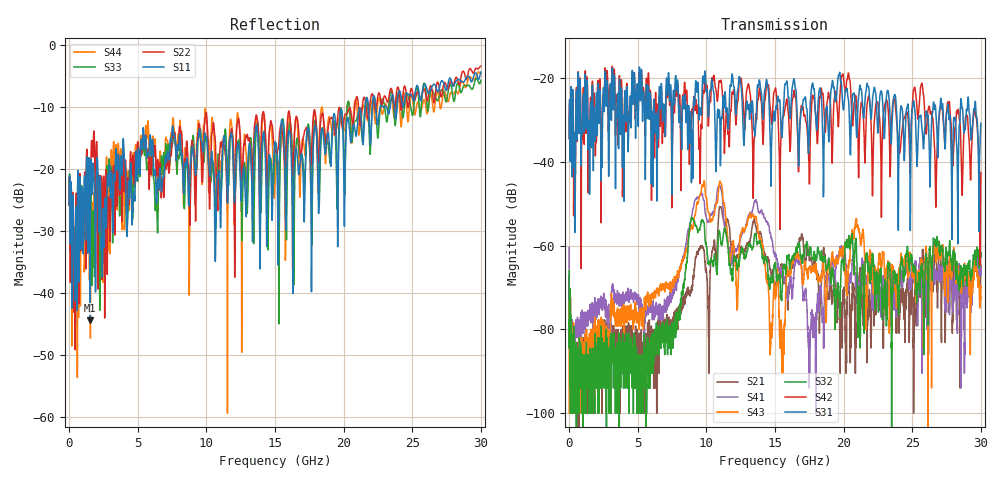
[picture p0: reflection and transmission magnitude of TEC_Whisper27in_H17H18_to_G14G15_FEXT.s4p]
! Tyco Electronics
! H17H18-G14G15_FEXT
!! PART DESCRIPTION: Whisper 27in Megtron 6 VLP-HVLP-VLP Channel Model, bulkhead 2.4mm test pts
!! MODEL DESCRIPTION: System 4-port S-parameter
!! MODEL STATUS: Measured
!! MODEL GEOMETRY: Channel Model
!! MODEL FREQUENCY RANGE: DC to 30.000 GHz in 10.000 MHz frequency steps
!! MODEL EDGE RATE LIMITATION: 12.500 ps (Using conservative 0.5/Fmax rule of thumb)
!! TIME-DOMAIN TRANSFORM CAUTIONS:
!! 1.) Do not simulate transient edge rates faster than the number listed above.  Edge rates faster than this number
!!  contain significant spectral content at frequencies above the model's highest frequency.
!! 2.) Even when simulating edge rates that are slower than the number listed above, be aware that the best time
!!  resolution possible with a direct iFFT is (1 / 2Fmax).  As a result, time resolution is typically not adequate
!!  for most time-domain simulations unless tricks such as windowing are used to minimize leakage and aliasing.
!! 3.) Because the model has a uniform frequency step, a direct iFFT will result in an impulse that that has a time
!!  length given by either (1 / Fstep) or (1 / 2Fstep), depending on the transform being used.  Care has been taken
!!  in selecting the frequency step to ensure a settled impulse response for the model.  Therefore, convolution with
!!  the model's impulse response should present no issues.  However, if directly concatenating s-parameter models
!!  in the frequency domain a user must either interpolate necessary interim frequencies or complete impulse response
!!  zero-padding.  Impulse response zero-padding is more difficult, but more accurate.
!! PORT DEFINITIONS:
!! Port  1  ----->  Side A  H17  G14  Side B  <-----  Port  2
!! Port  3  ----->  Side A  H18  G15  Side B  <-----  Port  4
! Point-to-Point link (differential)  !
! Connectors:  !
!  1: STRADA Whisper  !
! Materials:  !
!  Backplane: Megtron-6 HVLP  !
!  Daughtercard: Megtron-6 VLP  !
! Stack-up:  !
!  Backplane: 20 layers, 200mil thick  !
!  Daughtercard: 14 layers, 110mil thick  !
! Trace Length:  !
!  Backplane: 17in  !
!  Daightercards: 5in  !
! Trace Width:  !
!  Backplane: 8-13-8 mils  !
!  Daughtercards: 6-9-6 mils  !
! Geometry:  !
!  Backplane: Stripline  !
!  Daughtercards: Stripline  !
! Freq. Range: 0 GHz - 30 GHz  !
! Note1: non-mixed-mode s-parameters  !
! Note2: channel includes 2.4mm test points  !
! Touchstone data converted from IdEM dataset
# GHz S MA R 50
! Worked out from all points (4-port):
!   3000 points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, 10 MHz to 30 GHz, reference 50 ohm
!   strongest paths, dB at 10 MHz, 7.51 GHz, 15.01 GHz, 22.51 GHz, 30 GHz:
!     S31: -34.4, -43.9, -30.2, -32.7, -30.8
!     S42: -34.5, -40.8, -22.7, -26.3, -42.6
!     S32: -66.0, -80.0, -64.9, -71.7, -62.7
!     S43: -73.2, -69.1, -71.4, -65.5, -69.6
!     S41: -60.4, -71.4, -62.6, -71.1, -66.9
!     S21: -67.1, -80.9, -69.6, -68.6, -64.7
!   lowest |S11| = -44.4 dB at 1.53 GHz (marker M1), VSWR 1.01, Z = 49.6 - j0.456 ohm
!   |S11| at or under -10 dB: start of sweep to 21.58 GHz; 21.81 GHz to 22.09 GHz (281.3 MHz wide, 1.28 % of centre); 22.34 GHz to 22.68 GHz (341.6 MHz wide, 1.52 % of centre)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
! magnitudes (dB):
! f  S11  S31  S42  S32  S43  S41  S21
! 10 MHz  -25.6  -34.4  -34.5  -66.0  -73.2  -60.4  -67.1
! 1.53 GHz  -44.4  -33.3  -28.8  -94.0  -84.4  -74.0  -94.0
! 7.51 GHz  -13.8  -43.9  -40.8  -80.0  -69.1  -71.4  -80.9
! 9.77 GHz  -17.3  -19.8  -23.0  -54.3  -46.0  -48.8  -60.4
! 15.48 GHz  -12.2  -33.3  -31.4  -72.0  -80.9  -65.8  -64.6
! 20.94 GHz  -14.5  -33.9  -26.2  -60.6  -53.8  -69.1  -69.6
! 30 GHz  -4.4  -30.8  -42.6  -62.7  -69.6  -66.9  -64.7
